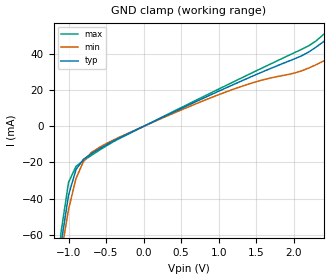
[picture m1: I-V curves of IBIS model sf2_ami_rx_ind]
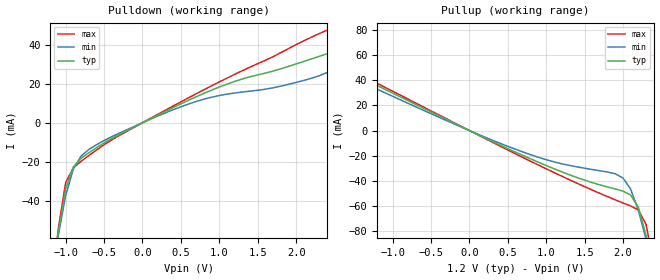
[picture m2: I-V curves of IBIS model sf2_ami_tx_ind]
|   Microsemi Corporation
|   SmarFusion2/IGLOO2 Industrial IBIS-AMI Models
[IBIS ver]   5.0
[File name]   sf2_igl2_ami_ind.ibs
[File Rev]   1.3
[Date]   February 1, 2019
[Disclaimer] These IBIS Models are Provided "As is" with NO WARRANTY
   whatsoever and signal integrity software specifically disclaims any
   implied warranties of merchantability, fitness for a particular
   purpose or against infringement.
[Source]   Original model developed in collaboration with Sigrity. Optimized by SiSoft.
[Notes]   Known limitations: Main tap is limited to maximum amplitude setting only
   and cannot be adjusted.
-Revision History:
1.4: February 1, 2019
   * Added model limitation note on abicdr_tx.ami and sf2_igl2_ami_ind.ibs files.
1.3: July 22, 2015
   * Added Algorithmic Model to support 64-bit Window environment
1.2: April 2, 2015
   * Added new RLC packages in Package section.
1.1: June 12, 2014
   * Updated Package section.
   * Consolidated the IGLOO2 and SmartFusion2 IBIS AMI Model
   * Updated the RX .ami model to clarify comments.
1.05: 6 November 2013
   Based on the model 1.0 model supplied by Microsemi dated 18 March 2013.
   This model has been optimized for use with SiSoft's QCD Simulator. Points of note:
   * Updated [Ramp] data to correct single-ended / differential issues
   * Updated C_comp values using data provided by Microsemi
   * Updated TX .ami file to disable auto EQ mode (does not work with QCD)
   * Included TX jitter data derived from PCIe Gen2 compliance testing
   * Signed models as QCD Certified
1.0: 18 March 2013 20:52:13
   * Original model supplied by Microsemi
[Copyright]  (c) 2014, Microsemi Corporation, All Rights Reserved.
[Component]  SF2_IGL2_ibis_ami_ind
[Manufacturer] Microsemi Corporation
[Package]
|   typ   min   max
| M2S/M2GL005
|R_pkg   0.72029   0.51528   1.0002   |005-FG484
|L_pkg   5.797e-9   4.155e-9   8.073e-9   |005-FG484
|C_pkg   1.116e-12   7.907e-13   1.753e-12   |005-FG484
|R_pkg   0.27009   0.041405   0.45769   |005-VF256
|L_pkg   4.091e-9   8.144e-10   7.139e-9   |005-VF256
|C_pkg   9.403e-13   6.174e-13   2.852e-12   |005-VF256
|R_pkg   0.47234   0.051444   0.70881   |005-VF400
|L_pkg   3.73e-9   4.383e-10   5.254e-9   |005-VF400
|C_pkg   9.092e-13   5.433e-13   3.219e-12   |005-VF400
|R_pkg   0.45289   0.15933   0.53232   |005-TQ144
|L_pkg   7.371e-9   3.475e-9   8.58e-9   |005-TQ144
|C_pkg   5.58e-13   4.777e-13   2.009e-12   |005-TQ144
| M2S/M2GL010
|R_pkg   0.66635   0.053835   1.0211   |010-FG484
|L_pkg   5.248e-9   6.178e-10   7.432e-9   |010-FG484
|C_pkg   1.306e-12   8.624e-13   3.748e-12   |010-FG484
|R_pkg   0.45429   0.057027   0.75756   |010-VF256
|L_pkg   3.996e-9   5.786e-10   5.727e-9   |010-VF256
|C_pkg   7.828e-13   3.988e-13   2.733e-12   |010-VF256
|R_pkg   0.42093   0.053275   0.67244   |010-VF400
|L_pkg   3.621e-9   5.054e-10   5.523e-9   |010-VF400
|C_pkg   1.012e-12   7.358e-13   4.005e-12   |010-VF400
|R_pkg   1.0678   0.95825   1.2776   |010-TQ144
|L_pkg   6.828e-9   5.979e-9   8.176e-9   |010-TQ144
|C_pkg   5.261e-13   4.459e-13   6.909e-13   |010-TQ144
| M2S/M2GL025
|R_pkg   0.62161   0.045855   0.88864   |025-FG484
|L_pkg   4.896e-9   4.955e-10   6.635e-9   |025-FG484
|C_pkg   1.283e-12   7.336e-13   4.781e-12   |025-FG484
|R_pkg   0.5113   0.081888   0.79004   |025-VF256
|L_pkg   4.3e-9   8.149e-10   6.356e-9   |025-VF256
|C_pkg   9.84e-13   5.422e-13   3.998e-12   |025-VF256
|R_pkg   0.56911   0.07806   0.87745   |025-VF400
|L_pkg   4.165e-9   7.124e-10   5.915e-9   |025-VF400
|C_pkg   1.037e-12   6.508e-13   4.436e-12   |025-VF400
|R_pkg   0.98263   0.44871   1.4996   |025-FCS325
|L_pkg   2.992e-9   1.127e-9   4.449e-9   |025-FCS325
|C_pkg   7.686e-13   4.28e-13   1.093e-12   |025-FCS325
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R_pkg   0.65025   0.050477   0.98075   |050-FG896
L_pkg   8.654e-9   4.198e-9   1.391e-8   |050-FG896
C_pkg   1.881e-12   1.117e-12   7.153e-12   |050-FG896
|R_pkg   0.64708   0.10714   1.1617   |050-FG484
|L_pkg   4.885e-9   8.618e-10   8.001e-9   |050-FG484
|C_pkg   1.224e-12   7.009e-13   2.089e-12   |050-FG484
|R_pkg   0.51212   0.082442   0.77494   |050-VF400
|L_pkg   3.938e-9   7.719e-10   5.981e-9   |050-VF400
|C_pkg   9.187e-13   5.253e-13   3.26e-12   |050-VF400
|R_pkg   0.87592   0.4729   1.2989   |050-FCS325
|L_pkg   2.542e-9   1.291e-9   3.732e-9   |050-FCS325
|C_pkg   6.621e-13   4.118e-13   9.479e-13   |050-FCS325
| M2S/M2GL060
|R_pkg   0.58359   0.09068   0.74939   |060-FG676
|L_pkg   5.269e-9   9e-10   6.659e-9   |060-FG676
|C_pkg   1.37e-12   5.634e-13   4.553e-12   |060-FG676
|R_pkg   0.56892   0.053004   0.79188   |060-FG484
|L_pkg   4.842e-9   5.148e-10   6.754e-9   |060-FG484
|C_pkg   1.575e-12   9.705e-13   7.459e-12   |060-FG484
|R_pkg   0.52053   0.072609   0.81109   |060-VF400
|L_pkg   4.301e-9   6.587e-10   6.035e-9   |060-VF400
|C_pkg   7.921e-13   3.769e-13   2.744e-12   |060-VF400
|R_pkg   0.8976   0.13778   1.274   |060-FCS325
|L_pkg   2.041e-9   3.18e-10   3.117e-9   |060-FCS325
|C_pkg   8.765e-13   4.713e-13   3.781e-12   |060-FCS325
| M2S/M2GL090
|R_pkg   0.63738   0.081807   0.76878   |090-FG676
|L_pkg   4.82e-9   7.761e-10   6.16e-9   |090-FG676
|C_pkg   1.49e-12   1.064e-12   7.809e-12   |090-FG676
|R_pkg   0.64363   0.064239   0.93501   |090-FG484
|L_pkg   4.937e-9   6.079e-10   6.828e-9   |090-FG484
|C_pkg   1.588e-12   6.307e-13   1.263e-11   |090-FG484
|R_pkg   0.82801   0.25425   1.2469   |090-FCS325
|L_pkg   2.074e-9   7.125e-10   3.565e-9   |090-FCS325
|C_pkg   9.158e-13   3.94e-13   1.405e-12   |090-FCS325
| M2S/M2GL150
|R_pkg   0.67258   0.11704   1.2705   |150-FCV484
|L_pkg   3.013e-9   9.675e-10   4.881e-9   |150-FCV484
|C_pkg   1.45e-12   7.195e-13   2.327e-12   |150-FCV484
|R_pkg   0.46246   0.10876   0.7535   |150-FCS536
|L_pkg   1.775e-9   4.138e-10   2.986e-9   |150-FCS536
|C_pkg   9.306e-13   4.484e-13   5.765e-12   |150-FCS536
|R_pkg   0.86225   0.11212   1.7907   |150-FC1152
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[Pin]   signal_name   model_name   R_pin  L_pin  C_pin
1p   sf2_tx_p   sf2_ami_tx_ind   NA   NA   NA
1n   sf2_tx_n   sf2_ami_tx_ind   NA   NA   NA
2p   sf2_rx_p   sf2_ami_rx_ind   NA   NA   NA
2n   sf2_rx_n   sf2_ami_rx_ind   NA   NA   NA
[Diff_Pin] inv_pin vdiff tdelay_typ tdelay_min tdelay_max
1p   1n   0.1V  NA   NA   NA
2p   2n   0.1V  NA   NA   NA
| Models and submodels in the file (2): sf2_ami_rx_ind (Input), sf2_ami_tx_ind (Output)
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|   Model sf2_ami_rx_ind
[Model] sf2_ami_rx_ind
|SiSoft ModelSignature1 3d05c4ffd32297e9a56824a110eab5edba11344b8333c9be1fca2d676f9db396 Certified
Model_type Input
C_comp 0.914p 0.471p 1.37p
Vinh = 0.55
Vinl = 0.45
| Differential package model for post-route analysis
|SiSoft Diff_Package SF2_FG896_472673AP0A_0308_PCIE2_TxRx.s4p.smod s_SF2_FG896_472673AP0A_0308_PCIE2_TxRx
[Algorithmic Model]
Executable Windows_VisualStudio7.1.3088_32 abicdr_rx.dll   abicdr_rx.ami
Executable Windows_VisualStudio7.1.3088_64 abicdr_x64_rx.dll  abicdr_rx.ami
Executable Linux_gcc3.2.3_64   abicdr_rh64_rx.dll abicdr_rx.ami
[End Algorithmic Model]
[Temperature Range]   25C   100C   -40C
[Voltage Range]   1.2V   1.14V   1.26V
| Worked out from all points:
|   GND clamp passes 1 mA (typ) near -0.05 V on its own axis
[GND Clamp]
|Voltage   I(typ)   I(min)   I(max)
-2.5V     -710.8mA   -586mA     -917.4mA
-1.2V     -101.9mA   -101.4mA   -104.9mA
-1.1V     -65.27mA   -71.02mA   -58.74mA
-1V       -38.09mA   -45.93mA   -31.05mA
-900mV    -23.87mA   -28.79mA   -22.1mA
-800mV    -18.2mA    -19.37mA   -18.94mA
-700mV    -15.32mA   -14.63mA   -16.19mA
-600mV    -12.78mA   -11.89mA   -13.5mA
200mV     3.966mA    3.674mA    4.161mA
1.1V      21.34mA    19.1mA     22.67mA
2.2V      41.17mA    32.28mA    44.62mA
2.5V      50.17mA    38.38mA    55.08mA
|   Model sf2_ami_tx_ind
[Model] sf2_ami_tx_ind
|SiSoft ModelSignature1 ab2bd8164ee5c105ce34143a7b87f5e1272386a81d776afbbc55d70f50a38479 Certified
Model_type Output
C_comp 0.914p 0.471p 1.37p
Cref = 0
Vref = 0.5
Rref = 50
Vmeas = 0.6
| Differential package model for post-route analysis
|SiSoft Diff_Package SF2_FG896_472673AP0A_0308_PCIE2_TxRx.s4p.smod s_SF2_FG896_472673AP0A_0308_PCIE2_TxRx
[Algorithmic Model]
Executable Windows_VisualStudio7.1.3088_32 abicdr_tx.dll   abicdr_tx.ami
Executable Windows_VisualStudio7.1.3088_64 abicdr_x64_tx.dll  abicdr_tx.ami
Executable Linux_gcc3.2.3_64   abicdr_rh64_tx.dll abicdr_tx.ami
[End Algorithmic Model]
[Temperature Range]   25C   100C   -40C
[Voltage Range]   1.2V   1.14V   1.26V
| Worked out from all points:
|   slope of the pulldown table from 0 to 0.18 V, typ, clamps not added: 50.4 ohm
|   slope of the pullup table from 0 to 0.18 V, typ, clamps not added: 34.2 ohm
[Pulldown]
|Voltage   I(typ)   I(min)   I(max)
-2.5V     -663.6mA   -536mA     -871.7mA
-1.2V     -90.34mA   -85.39mA   -97.87mA
-1.1V     -57.52mA   -58.72mA   -55.41mA
-1V       -33.95mA   -37.35mA   -30.72mA
-900mV    -22.69mA   -23.72mA   -23.1mA
-800mV    -18.27mA   -17.12mA   -19.81mA
-600mV    -12.82mA   -11.3mA    -14.02mA
100mV     1.995mA    1.749mA    2.168mA
700mV     13.31mA    10.9mA     14.86mA
1.2V      21.19mA    15.24mA    24.8mA
1.8V      27.64mA    18.75mA    35.91mA
2.5V      36.63mA    27.62mA    49.06mA
[Pullup]
|Voltage   I(typ)   I(min)   I(max)
-3.7V     173.4mA    160.1mA    190.7mA
-2.6V     83.25mA    81.33mA    83.4mA
-1.9V     57.14mA    53.41mA    59.48mA
100mV     -2.937mA   -2.611mA   -3.126mA
1V        -27.86mA   -23.21mA   -30.45mA
1.9V      -46.55mA   -34.45mA   -55.2mA
2V        -48.22mA   -37.82mA   -57.66mA
2.1V      -51.37mA   -46.71mA   -60.05mA
2.2V      -61.31mA   -63.56mA   -63.28mA
2.3V      -83.51mA   -86.68mA   -74.79mA
2.4V      -114.9mA   -113.6mA   -106.5mA
3.6V      -622.5mA   -520.6mA   -794.4mA
[Ramp]
| variable   typ   min   max
dV/dt_r 0.3912/8.652e-11   0.3464/9.033e-11   0.4245/9.614e-11
dV/dt_f 0.3912/7.387e-11   0.3464/7.723e-11   0.4245/7.205e-11
R_load = 50
|End [Model] sf2_ami_tx_ind
|End [Component]
